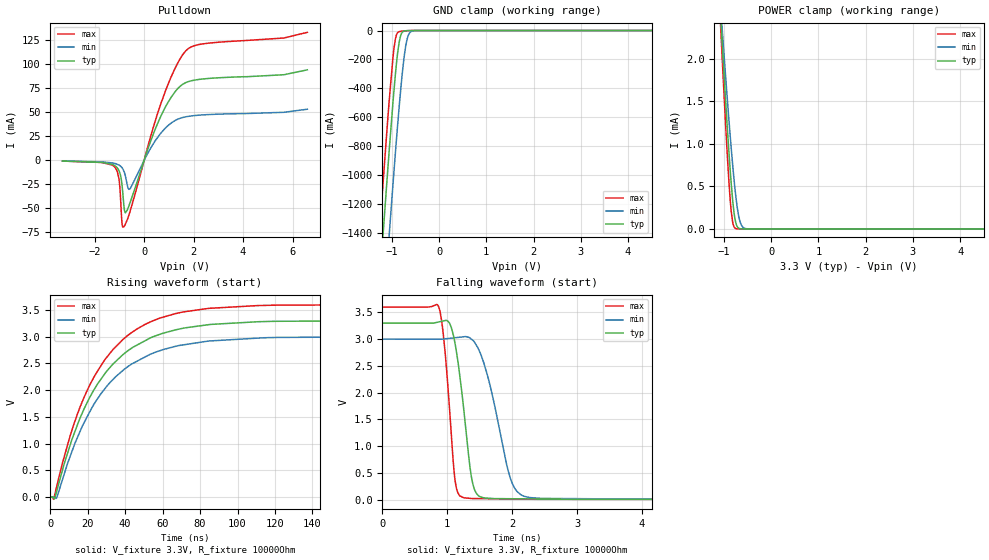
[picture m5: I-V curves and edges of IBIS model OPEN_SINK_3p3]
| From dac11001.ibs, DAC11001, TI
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|   OPEN_SINK_3p3 Model
[Model]   OPEN_SINK_3p3
Model_type   Open_sink
Polarity   Non-Inverting
Vmeas = 1.65
Vref = 3.3
Cref = 2pF
Rref = 10000
|   typ   min   max
C_comp   0.902pF   0.882pF   0.903pF
[Voltage Range]   3.3   3   3.6
[Temperature Range]   25   125   -40
[Pullup Reference]   3.3   3   3.6
[Pulldown Reference]   0   0   0
[Power Clamp Reference]   3.3   3   3.6
[GND Clamp Reference]   0   0   0
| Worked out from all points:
|   slope of the pulldown table from 0 to 0.495 V, typ, clamps not added: 14 ohm
|   GND clamp passes 1 mA (typ) near -0.68 V on its own axis
|   POWER clamp passes 1 mA (typ) near -0.90 V on its own axis
|   falling waveform, V_fixture 3.3V, R_fixture 10000Ohm: 20-80 % time 187ps typ, 325ps min, 135ps max; typ from 3.3 V to 0.004 V
|   rising waveform, V_fixture 3.3V, R_fixture 10000Ohm: 20-80 % time 30.3ns typ, 31ns min, 29.8ns max; typ from 0.004 V to 3.3 V
[Pulldown]
|   Voltage   I(typ)   I(min)   I(max)
-3.3V     -726uA     -595.1uA   -699.9uA
-1.191V   -5.393mA   -3.19mA    -6.875mA
-1.023V   -10.33mA   -4.81mA    -18.55mA
-943.8mV  -16.9mA    -6.252mA   -43.98mA
-884.4mV  -27.86mA   -7.971mA   -67.6mA
-815.1mV  -48.31mA   -11.34mA   -69.15mA
-755.7mV  -54.62mA   -16.42mA   -66.26mA
-577.5mV  -44.7mA    -29.79mA   -53.9mA
660mV     45.17mA    27.86mA    57.83mA
1.264V    71.95mA    41.74mA    96.68mA
1.68V     81.06mA    45.42mA    114.1mA
6.6V      94.43mA    53.35mA    133.5mA
[GND Clamp]
|   Voltage   I(typ)   I(min)   I(max)
-3.3V     -11.71A    -12.27A    -11.39A
-1.251V   -1.713A    -2.306A    -1.357A
-1.181V   -1.393A    -1.985A    -1.038A
-1.053V   -818.2mA   -1.401A    -474.3mA
-953.7mV  -412mA     -969.6mA   -122.1mA
-904.2mV  -236.7mA   -763.2mA   -32.34mA
-844.8mV  -80.92mA   -529.1mA   -8.148mA
-795.3mV  -20.6mA    -351.8mA   -4.81mA
-706.2mV  -1.632mA   -108.6mA   -1.977mA
-646.8mV  -462.8uA   -30.49mA   -818.4uA
-557.7mV  -68.68uA   -2.742mA   -121.7uA
6.6V      0A         0A         0A
[POWER Clamp]
|   Voltage   I(typ)   I(min)   I(max)
-3.3V     25.93mA    21.68mA    29.86mA
-1.063V   2.441mA    2.558mA    2.309mA
-1.053V   2.346mA    2.481mA    2.197mA
-1.013V   1.969mA    2.173mA    1.757mA
-924mV    1.16mA     1.502mA    831.4uA
-874.5mV  752uA      1.15mA     401.8uA
-844.8mV  532.6uA    948.6uA    206.9uA
-815.1mV  342.4uA    758.1uA    82.55uA
-745.8mV  69.61uA    374.9uA    4.177uA
-656.7mV  3.216uA    84.12uA    47.43nA
-528mV    13.79nA    3.131uA    0A
6.6V      0A         0A         0A
[Ramp]
R_load = 10000
|   typ   min   max
dV/dt_r   1.97755/3.03031e-08   1.79657/3.09614e-08   2.15783/2.9634e-08
dV/dt_f   1.97755/1.86765e-10   1.79657/3.23484e-10   2.15783/1.3447e-10
[Falling Waveform]
V_fixture = 3.3V
V_fixture_min = 3V
V_fixture_max = 3.6V
R_fixture = 10000Ohm
C_fixture = 0F
|   Time   V(typ)   V(min)   V(max)
0s        3.3V       3V         3.6V
865.4ps   3.321V     2.999V     3.613V
962.9ps   3.347V     3.006V     2.803V
1.063ns   3.219V     3.019V     1.216V
1.185ns   2.39V      3.036V     79.16mV
1.35ns    602.8mV    3.021V     21.62mV
1.444ns   124.3mV    2.895V     17.29mV
2.006ns   14.38mV    288.9mV    9.489mV
2.399ns   10.21mV    25.6mV     4.047mV
3.5us     4.08mV     5.716mV    3.62mV
[Rising Waveform]
V_fixture = 3.3V
V_fixture_min = 3V
V_fixture_max = 3.6V
R_fixture = 10000Ohm
C_fixture = 0F
|   Time   V(typ)   V(min)   V(max)
0s        4.08mV     5.716mV    3.62mV
1.826ns   -13.57mV   2.118mV    -37.16mV
3.434ns   111.6mV    -11.98mV   197.6mV
10.94ns   1.008V     791.3mV    1.182V
19.79ns   1.774V     1.507V     2.001V
28.29ns   2.265V     1.987V     2.525V
38.85ns   2.664V     2.369V     2.948V
66.86ns   3.126V     2.818V     3.43V
110.8ns   3.278V     2.972V     3.58V
3.5us     3.3V       3V         3.6V
